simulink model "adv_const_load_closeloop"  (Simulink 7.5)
settings: Solver=ode113  StartTime=0.0  StopTime=2  MaxStep=1e-4  MinStep=1e-5  RelTol=1e-5
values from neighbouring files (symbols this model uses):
  B = 0.0001    [adv1.m]    (also in adv1_plot_eaia.m; adv1_plot_te_speed.m; lookup01_plot.m; NEW_VAR .m)
  J = .0001    (= 0.0001)    [adv1.m]    (also in adv1_plot_eaia.m; adv1_plot_te_speed.m; lookup01_plot.m; NEW_VAR .m)
  kw = 0.0445    [adv1.m]    (also in adv1_plot_eaia.m; adv1_plot_te_speed.m; lookup01_plot.m = 0.0365; NEW_VAR .m)
  L = .00192    (= 0.00192)    [adv1.m]    (also in adv1_plot_eaia.m; adv1_plot_te_speed.m; lookup01_plot.m; NEW_VAR .m)
  P = 4    [adv1.m]    (also in adv1_plot_eaia.m; adv1_plot_te_speed.m; lookup01_plot.m; NEW_VAR .m)
  R = 1.5    [adv1.m]    (also in adv1_plot_eaia.m; adv1_plot_te_speed.m; lookup01_plot.m; NEW_VAR .m)
  sp = 2500    [plot_advance0_2.m]    (also in plot_closeloop.m)
  T0 = 0.0001    [adv1.m]    (also in adv1_plot_eaia.m; adv1_plot_te_speed.m; lookup01_plot.m; NEW_VAR .m)
  W0 = 2    [adv1.m]    (also in adv1_plot_eaia.m; adv1_plot_te_speed.m; lookup01_plot.m; NEW_VAR .m)

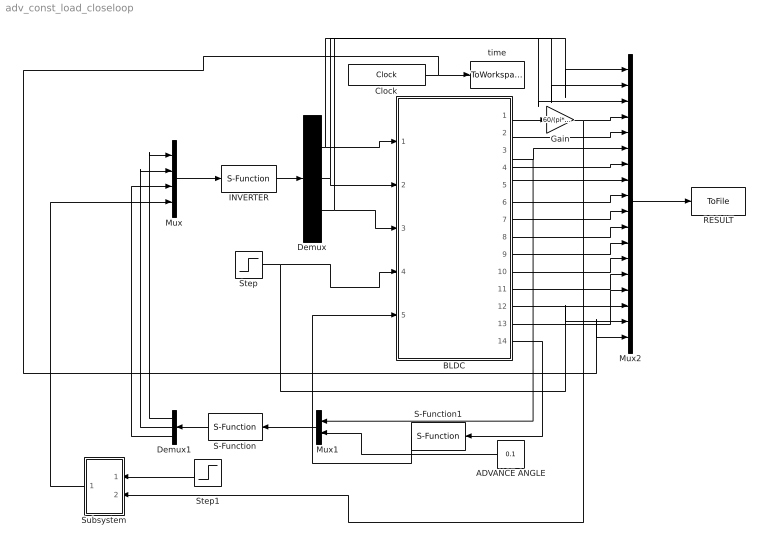
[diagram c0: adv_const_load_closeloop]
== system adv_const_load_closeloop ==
  ADVANCE ANGLE : Constant  Value=0.1  OutDataType=fixdt(1, 16)  OutScaling=2^0
  BLDC : Subsystem
  Clock : Clock
  Demux : Demux  Outputs=3
  Demux1 : Demux  Outputs=3
  Gain : Gain  Gain=60/(pi*P)  ParameterDataType=fixdt(1, 16)  ParameterScaling=2^0  OutDataType=fixdt(1, 16)  OutScaling=2^0
  INVERTER : S-Function  FunctionName=inverter  Parameters=vmax  EnableBusSupport=off  mask{vmax=24}
      mask prompts: vmax "maximum dc bus"
  Mux : Mux
  Mux1 : Mux  Inputs=2
  Mux2 : Mux  Inputs=18
  RESULT : ToFile  Filename=bldc_advangle
  S-Function : S-Function  FunctionName=BLDC_adv_2in  Parameters=angle  EnableBusSupport=off  mask{angle=0}
      mask prompts: angle "advance  angle"
  S-Function1 : S-Function  FunctionName=sam_adv_ktc  Parameters=R,L,J,P,kw  EnableBusSupport=off
  Step : Step  After=.1  SampleTime=0
  Step1 : Step  After=sp  SampleTime=0
  Subsystem : Subsystem
  time : ToWorkspace  VariableName=time  SampleTime=-1  SaveFormat=Array
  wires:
  INVERTER/1 -> Demux/1
  Mux/1 -> INVERTER/1
  BLDC/1(W) -> Gain/1
  Clock/1 -> time/1, Mux2/18
  S-Function/1 -> Demux1/1
  BLDC/14(outadv) -> S-Function1/1
  Mux1/1 -> S-Function/1
  BLDC/3(Phi) -> Mux1/1, Mux2/6
  S-Function1/1 -> BLDC/5(inadv)
  Demux/1 -> BLDC/1(Va), Mux2/1
  Demux/2 -> BLDC/2(Vb), Mux2/2
  Demux/3 -> BLDC/3(Vc), Mux2/3
  Demux1/1 -> Mux/1
  Demux1/2 -> Mux/2
  Demux1/3 -> Mux/3
  ADVANCE ANGLE/1 -> Mux1/2
  Gain/1 -> Mux2/4, Subsystem/2(pv)
  BLDC/2(Te) -> Mux2/5
  BLDC/4(HA) -> Mux2/7
  BLDC/5(HB) -> Mux2/8
  BLDC/6(HC) -> Mux2/9
  BLDC/7(ea) -> Mux2/10
  BLDC/8(eb) -> Mux2/11
  BLDC/9(ec) -> Mux2/12
  BLDC/10(theta) -> Mux2/13
  BLDC/11(ic) -> Mux2/14
  BLDC/12(ib) -> Mux2/15
  BLDC/13(ia) -> Mux2/16
  Mux2/1 -> RESULT/1
  Step/1 -> BLDC/4(Tload), Mux2/17
  Subsystem/1(Out1) -> Mux/4
  Step1/1 -> Subsystem/1(SP)

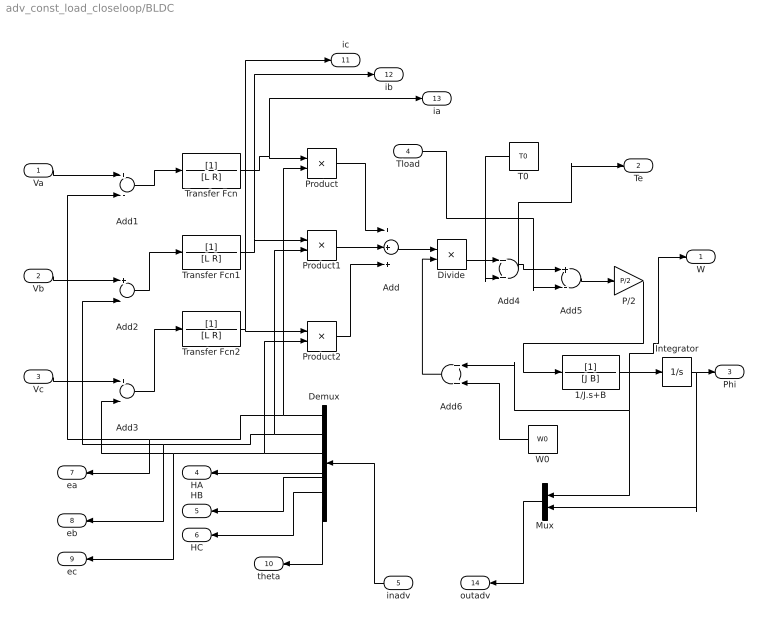
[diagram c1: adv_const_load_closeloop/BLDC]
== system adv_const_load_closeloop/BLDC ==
  Va : Inport  OutDataType=fixdt(1, 16)  OutScaling=2^0
  Vb : Inport  Port=2  OutDataType=fixdt(1, 16)  OutScaling=2^0
  Vc : Inport  Port=3  OutDataType=fixdt(1, 16)  OutScaling=2^0
  Tload : Inport  Port=4  OutDataType=fixdt(1, 16)  OutScaling=2^0
  inadv : Inport  Port=5  OutDataType=fixdt(1, 16)  OutScaling=2^0
  1/J.s+B : TransferFcn  Denominator=[J B]
  Add : Sum  Inputs=+++  OutDataType=fixdt(1, 16)  OutScaling=2^-10
  Add{1..3,5} (4 alike) : Sum  Inputs=+-  OutDataType=fixdt(1, 16)  OutScaling=2^-10
  Add4 : Sum  OutDataType=fixdt(1, 16)  OutScaling=2^-10
  Add6 : Sum  OutDataType=fixdt(1, 16)  OutScaling=2^-10
  Demux : Demux  Outputs=7
  Divide : Product  Inputs=*/  OutDataType=fixdt(1, 16)  OutScaling=2^-10
  Integrator : Integrator
  Mux : Mux  Inputs=2
  P/2 : Gain  Gain=P/2  ParameterDataType=fixdt(1, 16)  ParameterScaling=2^0  OutDataType=fixdt(1, 16)  OutScaling=2^0
  Product : Product  OutDataType=fixdt(1, 16)  OutScaling=2^0
  Product1 : Product  OutDataType=fixdt(1, 16)  OutScaling=2^0
  Product2 : Product  OutDataType=fixdt(1, 16)  OutScaling=2^0
  T0 : Constant  Value=T0  OutDataType=fixdt(1, 16)  OutScaling=2^0
  Transfer Fcn : TransferFcn  Denominator=[L R]
  Transfer Fcn1 : TransferFcn  Denominator=[L R]
  Transfer Fcn2 : TransferFcn  Denominator=[L R]
  W0 : Constant  Value=W0  OutDataType=fixdt(1, 16)  OutScaling=2^0
  W : Outport  OutDataType=fixdt(1, 16)  OutScaling=2^0
  Te : Outport  Port=2  OutDataType=fixdt(1, 16)  OutScaling=2^0
  Phi : Outport  Port=3  OutDataType=fixdt(1, 16)  OutScaling=2^0
  HA : Outport  Port=4  OutDataType=fixdt(1, 16)  OutScaling=2^0
  HB : Outport  Port=5  OutDataType=fixdt(1, 16)  OutScaling=2^0
  HC : Outport  Port=6  OutDataType=fixdt(1, 16)  OutScaling=2^0
  ea : Outport  Port=7  OutDataType=fixdt(1, 16)  OutScaling=2^0
  eb : Outport  Port=8  OutDataType=fixdt(1, 16)  OutScaling=2^0
  ec : Outport  Port=9  OutDataType=fixdt(1, 16)  OutScaling=2^0
  theta : Outport  Port=10  OutDataType=fixdt(1, 16)  OutScaling=2^0
  ic : Outport  Port=11  OutDataType=fixdt(1, 16)  OutScaling=2^0
  ib : Outport  Port=12  OutDataType=fixdt(1, 16)  OutScaling=2^0
  ia : Outport  Port=13  OutDataType=fixdt(1, 16)  OutScaling=2^0
  outadv : Outport  Port=14  OutDataType=fixdt(1, 16)  OutScaling=2^0
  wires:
  Add1/1 -> Transfer Fcn/1
  Add2/1 -> Transfer Fcn1/1
  Add3/1 -> Transfer Fcn2/1
  Transfer Fcn/1 -> Product/1, ia/1
  Transfer Fcn1/1 -> Product1/1, ib/1
  Transfer Fcn2/1 -> Product2/1, ic/1
  Demux/1 -> Add1/2, ea/1, Product/2
  Demux/2 -> Product1/2, Add2/2, eb/1
  Va/1 -> Add1/1
  Vb/1 -> Add2/1
  Vc/1 -> Add3/1
  Demux/3 -> Product2/2, Add3/2, ec/1
  Product/1 -> Add/1
  Product1/1 -> Add/2
  Product2/1 -> Add/3
  Add/1 -> Divide/1
  Add5/1 -> P/2/1
  Divide/1 -> Add4/1
  T0/1 -> Add4/2
  Add4/1 -> Add5/1, Te/1
  Tload/1 -> Add5/2
  P/2/1 -> 1/J.s+B/1
  1/J.s+B/1 -> Integrator/1, W/1, Add6/1, Mux/1
  Add6/1 -> Divide/2
  W0/1 -> Add6/2
  Integrator/1 -> Phi/1, Mux/2
  Demux/4 -> HA/1
  Demux/5 -> HB/1
  Demux/6 -> HC/1
  Demux/7 -> theta/1
  inadv/1 -> Demux/1
  Mux/1 -> outadv/1

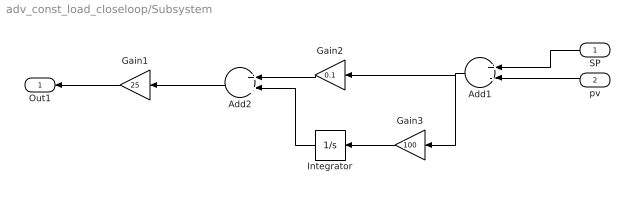
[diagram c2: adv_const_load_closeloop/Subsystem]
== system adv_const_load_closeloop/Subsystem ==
  SP : Inport  OutDataType=fixdt(1, 16)  OutScaling=2^0
  pv : Inport  Port=2  OutDataType=fixdt(1, 16)  OutScaling=2^0
  Add1 : Sum  Inputs=+-  OutDataType=fixdt(1, 16)  OutScaling=2^-10
  Add2 : Sum  OutDataType=fixdt(1, 16)  OutScaling=2^-10
  Gain1 : Gain  Gain=25  ParameterDataType=fixdt(1, 16)  ParameterScaling=2^0  OutDataType=fixdt(1, 16)  OutScaling=2^0
  Gain2 : Gain  Gain=0.1  ParameterDataType=fixdt(1, 16)  ParameterScaling=2^0  OutDataType=fixdt(1, 16)  OutScaling=2^0
  Gain3 : Gain  Gain=100  ParameterDataType=fixdt(1, 16)  ParameterScaling=2^0  OutDataType=fixdt(1, 16)  OutScaling=2^0
  Integrator : Integrator
  Out1 : Outport  OutDataType=fixdt(1, 16)  OutScaling=2^0
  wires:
  Add1/1 -> Gain2/1, Gain3/1
  Gain2/1 -> Add2/1
  Integrator/1 -> Add2/2
  Gain3/1 -> Integrator/1
  Add2/1 -> Gain1/1
  SP/1 -> Add1/1
  pv/1 -> Add1/2
  Gain1/1 -> Out1/1
